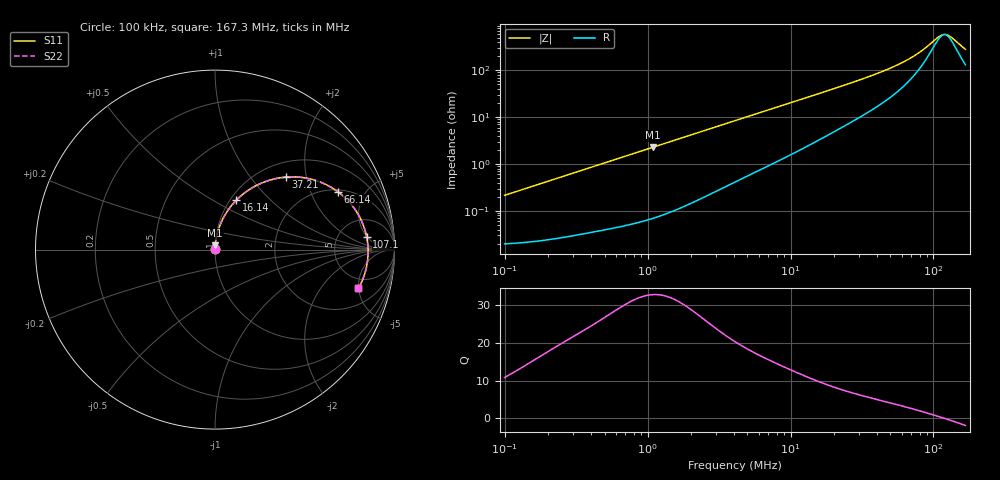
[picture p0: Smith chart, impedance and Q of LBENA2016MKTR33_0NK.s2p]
! LBENA2016MKTR33_0NK  S-PARAMETER MODEL  ( General Type )
! Model Generated by TAIYO YUDEN Corporation (http://www.ty-top.com)
! Version 1.0
! TAIYO YUDEN Control No. 211203
! Copyright(c) 2021 TAIYO YUDEN CO.,LTD. All Rights Reserved.
! Product Description (link to TY-COMPAS)
! https://ds.yuden.co.jp/TYCOMPAS/or/detail?pn=LBENA2016MKTR33M0NK&u=M
! Products Name : Inductors
! Characteristics :
!  Inductance : 0.33 uH , SRF(min) : -Hz , DC Resistance(max) : 0.022 Ohm
!  Rated Current : Saturation :5400 mA , Temp Rise : 4900 mA
!  Case Size : 2.0 x 1.6 / 0.079 x 0.063 [mm/inch] , Thickness : 1.2 / 0.047 [mm/inch]
!  (Conditions: Temperature = 25 degC , DC Bias Current/Voltage = 0A / 0V)
! External Node Assignments :
!  1  o---GGG---o  2
! GND o---------o GND
! Frequency Range : 0.1MHz  -  167.251077MHz  [ 402 STEP ]
# MHz S RI R 50
! Freq[MHz].  S11 Real  S11 Imag  S21 Real  S21 Imag  S12 Real  S12 Imag  S22 Real  S22 Imag
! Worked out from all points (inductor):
!   401 points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, 100 kHz to 167.3 MHz, reference 50 ohm
!   read as one part in series: L = 341 nH near 103.8 kHz
!   highest Q = 32.8 at 1.095 MHz (marker M1), where L = 333 nH
!   self-resonance near 119.2 MHz
!   S11 on the Smith chart (normalised r, x): 100 kHz: 1.00, +0.00; 16.14 MHz: 1.07, +0.65; 37.21 MHz: 1.29, +1.53; 66.14 MHz: 2.11, +3.19; 107.1 MHz: 10, +5; 167.3 MHz: 3.62, -4.97
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0.1  0.000202 0.00214  0.9998 -0.00214  0.9998 -0.00214  0.000202 0.00214
0.346668  0.000373 0.00735  0.9996 -0.00735  0.9996 -0.00735  0.000373 0.00735
1.095309  0.00122 0.0229  0.9988 -0.0229  0.9988 -0.0229  0.00122 0.0229
1.20179  0.0014 0.0251  0.9986 -0.0251  0.9986 -0.0251  0.0014 0.0251
2.343861  0.00416 0.0484  0.9958 -0.0484  0.9958 -0.0484  0.00416 0.0484
4.166227  0.0114 0.0843  0.9886 -0.0843  0.9886 -0.0843  0.0114 0.0843
8.432628  0.0393 0.162  0.9607 -0.162  0.9607 -0.162  0.0393 0.162
14.17747  0.0958 0.2503  0.9042 -0.2503  0.9042 -0.2503  0.0958 0.2503
16.14387  0.1188 0.2756  0.8812 -0.2756  0.8812 -0.2756  0.1188 0.2756
24.73725  0.2301 0.357  0.7699 -0.357  0.7699 -0.357  0.2301 0.357
37.20803  0.3952 0.4039  0.6048 -0.4039  0.6048 -0.4039  0.3952 0.4039
49.14881  0.5349 0.3926  0.4651 -0.3926  0.4651 -0.3926  0.5349 0.3926
57.01386  0.6123 0.3654  0.3877 -0.3654  0.3877 -0.3654  0.6123 0.3654
66.13751  0.6865 0.321  0.3135 -0.321  0.3135 -0.321  0.6865 0.321
82.63212  0.7809 0.2228  0.2191 -0.2228  0.2191 -0.2228  0.7809 0.2228
107.1437  0.8453 0.0697  0.1547 -0.0697  0.1547 -0.0697  0.8453 0.0697
113.2771  0.8508 0.0335  0.1492 -0.0335  0.1492 -0.0335  0.8508 0.0335
117.5598  0.8527 0.00914  0.1473 -0.00914  0.1473 -0.00914  0.8527 0.00914
126.6172  0.8522 -0.04  0.1478 0.04  0.1478 0.04  0.8522 -0.04
136.3723  0.8459 -0.0888  0.1541 0.0888  0.1541 0.0888  0.8459 -0.0888
161.1581  0.8108 -0.1939  0.1892 0.1939  0.1892 0.1939  0.8108 -0.1939
167.2511  0.7994 -0.2157  0.2006 0.2157  0.2006 0.2157  0.7994 -0.2157
